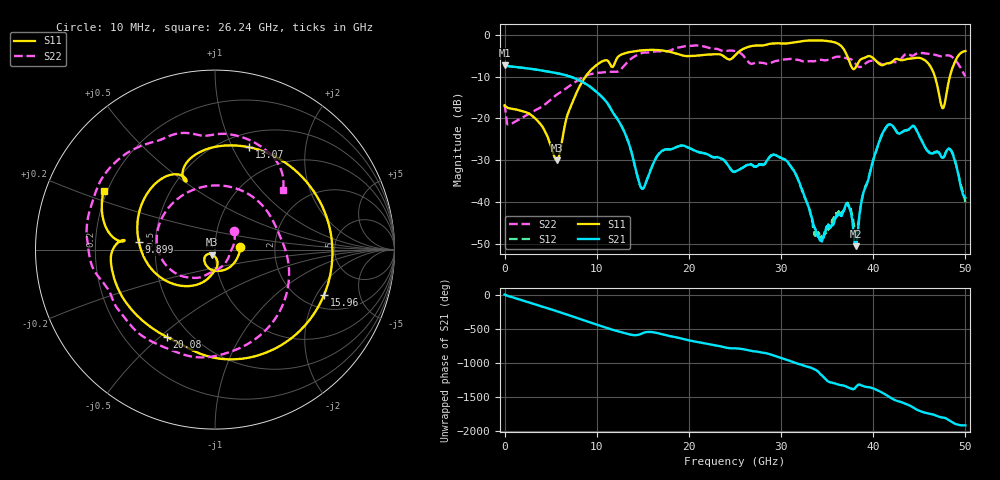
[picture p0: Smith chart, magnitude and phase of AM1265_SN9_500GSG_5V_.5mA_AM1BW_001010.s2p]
!Keysight Technologies,N5245B,MY58422270,A.16.20.02
!Date: Thursday, March 05, 2026 00:37:32
!Correction: S11(C  2-Port  )
!S21(C  2-Port  )
!S12(C  2-Port  )
!S22(C  2-Port  )
!S2P File: Measurements: S11, S21, S12, S22:
# Hz S  dB  R 50
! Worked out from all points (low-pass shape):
!   3201 points, 10 MHz to 50 GHz, reference 50 ohm
!   highest |S21| = -7.32 dB at 10 MHz (marker M1); lowest = -50.5 dB at 38.11 GHz (marker M2)
!   |S21| within 3 dB of the highest: start of sweep to 7.52 GHz
!   lowest |S11| = -30.0 dB at 5.665 GHz (marker M3), VSWR 1.07, Z = 48.5 - j2.71 ohm
!   |S11| at or under -10 dB: start of sweep to 8.795 GHz; 46.69 GHz to 48.31 GHz (1.621 GHz wide, 3.41 % of centre)
!   |S22| runs from -21.4 to -2.6 dB; largest |S21 - S12| = 0.0037
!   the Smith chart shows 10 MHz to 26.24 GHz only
!   S11 on the Smith chart (normalised r, x): 10 MHz: 1.33, +0.03; 9.899 GHz: 0.40, +0.04; 13.07 GHz: 0.65, +1.16; 15.96 GHz: 2.62, -2.32; 20.08 GHz: 0.37, -0.53; 26.24 GHz: 0.19, +0.24
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1e7  -16.94 4.8  -7.32 3.8  -7.39 3.6  -16.54 43.7
2.306416e9  -18.49 -87.3  -7.98 -97.6  -7.98 -97.7  -19.32 -78.3
5.665119e9  -30.02 -117.7  -9.18 118.8  -9.18 118.8  -14.33 -124.7
8.352081e9  -11.53 -129.9  -11.16 -3.4  -11.15 -3.4  -10.33 -171.6
9.898647e9  -7.40 174.3  -13.51 -74.3  -13.51 -74.3  -9.18 140.4
1.138272e10  -6.77 114.9  -17.12 -141.8  -17.11 -141.9  -8.86 70.0
1.306989e10  -4.42 71.7  -23.56 153.7  -23.53 153.9  -7.18 -19.3
1.483516e10  -3.75 12.4  -36.58 145.1  -36.57 144.9  -4.41 -94.7
1.595993e10  -3.64 -22.4  -31.71 171.6  -31.67 171.7  -4.10 -126.1
1.667854e10  -3.68 -43.4  -28.62 153.4  -28.66 153.7  -4.01 -142.3
2.008411e10  -5.10 -119.0  -27.10 46.8  -27.09 46.7  -2.71 159.5
2.5005e10  -4.96 173.6  -32.70 -68.4  -32.68 -68.5  -3.90 71.2
2.623913e10  -3.07 152.1  -31.19 -89.1  -31.18 -88.8  -5.92 41.5
3.048828e10  -2.11 80.8  -29.93 128.9  -30.05 128.6  -5.88 -49.3
3.334708e10  -1.38 35.5  -43.76 1.0  -44.00 4.6  -6.35 -127.9
3.667454e10  -3.07 -31.0  -42.69 107.0  -42.30 108.8  -5.35 165.4
3.811175e10  -7.74 -23.6  -50.49 81.3  -47.57 80.1  -7.04 139.4
4.167354e10  -6.83 -54.5  -21.43 -57.2  -21.54 -57.3  -6.82 114.3
4.509473e10  -5.58 -102.2  -24.56 87.1  -24.66 87.5  -4.34 75.0
4.653194e10  -9.00 -151.9  -28.27 36.1  -28.17 34.9  -4.72 53.8
4.770358e10  -16.91 70.3  -29.12 -11.1  -28.94 -11.7  -5.03 40.6
5e10  -3.91 -73.3  -38.95 -123.2  -39.95 -128.2  -9.92 4.5
